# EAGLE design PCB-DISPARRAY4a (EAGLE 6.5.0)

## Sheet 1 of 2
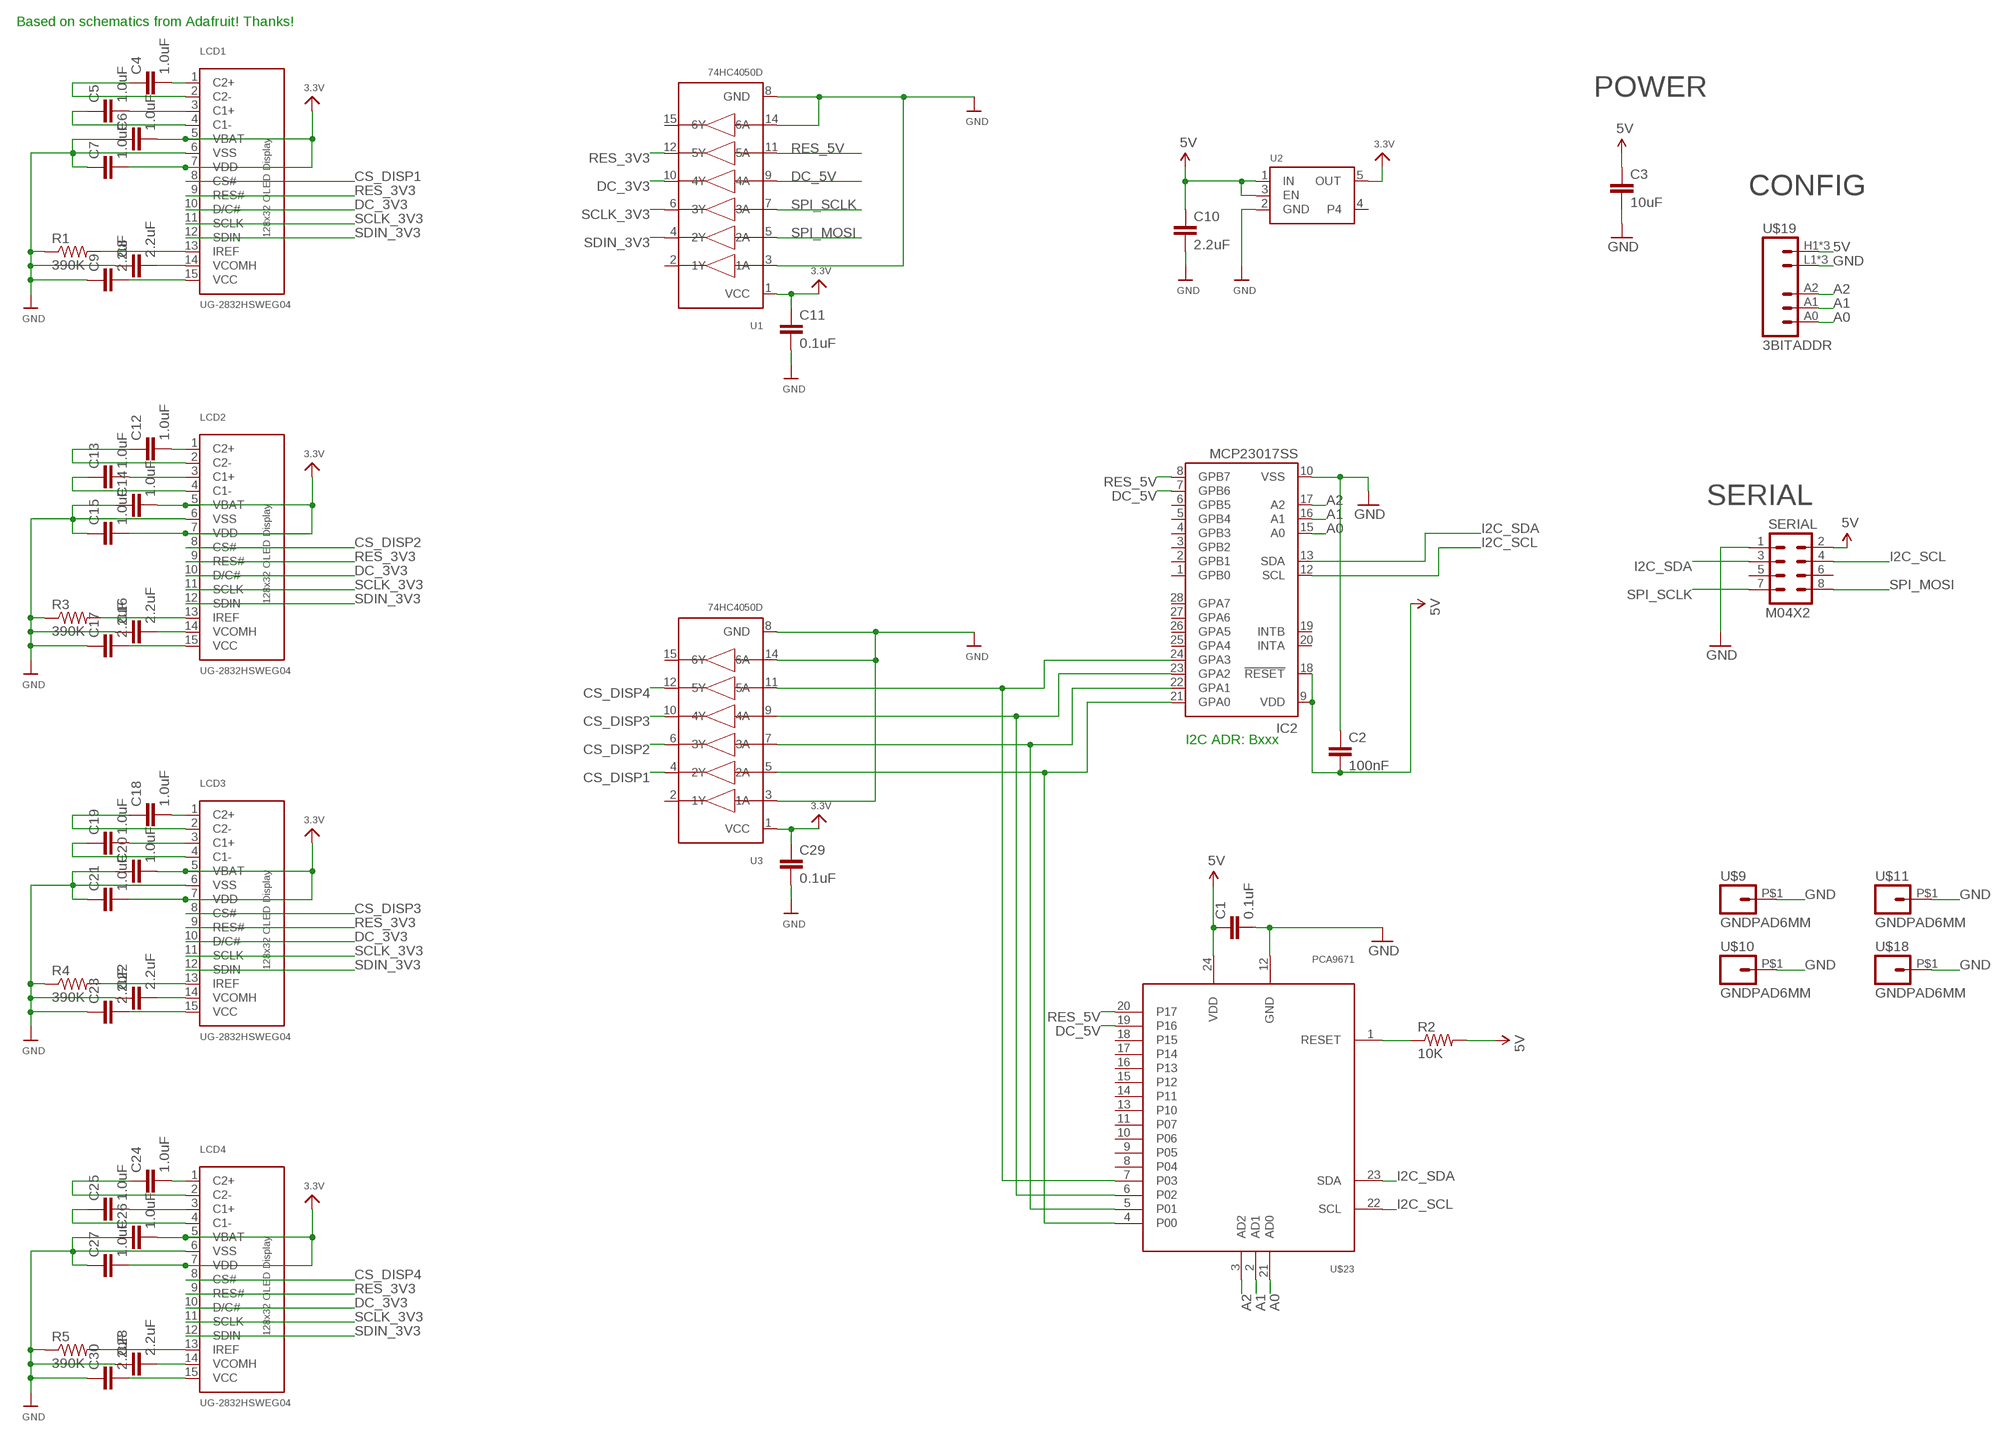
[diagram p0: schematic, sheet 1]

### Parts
C1  0.1uF  CAP0603-CAP  [0603-CAP]
C2  100nF  CAP0603-CAP  [0603-CAP]
C3  10uF  CAP0805  [0805]
C4  1.0uF  CAP0603-CAP  [0603-CAP]
C5  1.0uF  CAP0603-CAP  [0603-CAP]
C6  1.0uF  CAP0603-CAP  [0603-CAP]
C7  1.0uF  CAP0603-CAP  [0603-CAP]
C8  2.2uF  CAP0603-CAP  [0603-CAP]
C9  2.2uF  CAP0603-CAP  [0603-CAP]
C10  2.2uF  CAP0603-CAP  [0603-CAP]
C11  0.1uF  CAP0603-CAP  [0603-CAP]
C12  1.0uF  CAP0603-CAP  [0603-CAP]
C13  1.0uF  CAP0603-CAP  [0603-CAP]
C14  1.0uF  CAP0603-CAP  [0603-CAP]
C15  1.0uF  CAP0603-CAP  [0603-CAP]
C16  2.2uF  CAP0603-CAP  [0603-CAP]
C17  2.2uF  CAP0603-CAP  [0603-CAP]
C18  1.0uF  CAP0603-CAP  [0603-CAP]
C19  1.0uF  CAP0603-CAP  [0603-CAP]
C20  1.0uF  CAP0603-CAP  [0603-CAP]
C21  1.0uF  CAP0603-CAP  [0603-CAP]
C22  2.2uF  CAP0603-CAP  [0603-CAP]
C23  2.2uF  CAP0603-CAP  [0603-CAP]
C24  1.0uF  CAP0603-CAP  [0603-CAP]
C25  1.0uF  CAP0603-CAP  [0603-CAP]
C26  1.0uF  CAP0603-CAP  [0603-CAP]
C27  1.0uF  CAP0603-CAP  [0603-CAP]
C28  2.2uF  CAP0603-CAP  [0603-CAP]
C29  0.1uF  CAP0603-CAP  [0603-CAP]
C30  2.2uF  CAP0603-CAP  [0603-CAP]
IC2  MCP23017SS  [SSOP28]
LCD1  UG-2832HSWEG04  OLED_UG-2832HSWEG04WRAPAROUND  [UG-2832HSWEG04_WRAPAROUND]
LCD2  UG-2832HSWEG04  OLED_UG-2832HSWEG04WRAPAROUND  [UG-2832HSWEG04_WRAPAROUND]
LCD3  UG-2832HSWEG04  OLED_UG-2832HSWEG04WRAPAROUND  [UG-2832HSWEG04_WRAPAROUND]
LCD4  UG-2832HSWEG04  OLED_UG-2832HSWEG04WRAPAROUND  [UG-2832HSWEG04_WRAPAROUND]
R1  390K  RESISTOR0603-RES  [0603-RES]
R2  10K  RESISTOR0603-RES  [0603-RES]
R3  390K  RESISTOR0603-RES  [0603-RES]
R4  390K  RESISTOR0603-RES  [0603-RES]
R5  390K  RESISTOR0603-RES  [0603-RES]
SERIAL  M04X2  [2X4]
U1  74HC4050D  [SOIC16]
U2  VREG_SOT23-5  [SOT23-5]
U3  74HC4050D  [SOIC16]
U$9  GNDPAD6MM  [3.2MMPAD6MM]
U$10  GNDPAD6MM  [3.2MMPAD6MM]
U$11  GNDPAD6MM  [3.2MMPAD6MM]
U$18  GNDPAD6MM  [3.2MMPAD6MM]
U$19  3BITADDR  [3BITADDR]
U$23  PCA9671  [TSSOP24]

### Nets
3.3V: C6.2 C7.2 C11.1 C14.2 C15.2 C20.2 C21.2 C26.2 C27.2 C29.1 LCD1.5(VBAT) LCD1.7(VDD) LCD2.5(VBAT) LCD2.7(VDD) LCD3.5(VBAT) LCD3.7(VDD) LCD4.5(VBAT) LCD4.7(VDD) U1.1(VCC) U2.5(OUT) U3.1(VCC)
5V [Power]: C1.1 C2.2 C3.1 C10.1 IC2.9(VDD) IC2.18(!RESET) R2.2 SERIAL.2 U2.1(IN) U2.3(EN) U$19.H1(VCC) U$19.H2(VCC) U$19.H3(VCC) U$23.24(VDD)
A0: IC2.15(A0) U$19.A0 U$23.21(AD0)
A1: IC2.16(A1) U$19.A1 U$23.2(AD1)
A2: IC2.17(A2) U$19.A2 U$23.3(AD2)
CS_DISP1: LCD1.8(CS#) U3.4(2Y)
CS_DISP2: LCD2.8(CS#) U3.6(3Y)
CS_DISP3: LCD3.8(CS#) U3.10(4Y)
CS_DISP4: LCD4.8(CS#) U3.12(5Y)
DC_3V3: LCD1.10(D/C#) LCD2.10(D/C#) LCD3.10(D/C#) LCD4.10(D/C#) U1.10(4Y)
DC_5V: IC2.7(GPB6) U1.9(4A) U$23.19(P16)
GND [Power]: C1.2 C2.1 C3.2 C6.1 C7.1 C8.1 C9.1 C10.2 C11.2 C14.1 C15.1 C16.1 C17.1 C20.1 C21.1 C22.1 C23.1 C26.1 C27.1 C28.1 C29.2 C30.1 IC2.10(VSS) LCD1.6(VSS) LCD2.6(VSS) LCD3.6(VSS) LCD4.6(VSS) R1.1 R3.1 R4.1 R5.1 SERIAL.1 U1.3(1A) U1.8(GND) U1.14(6A) U2.2(GND) U3.3(1A) U3.8(GND) U3.14(6A) U$9.P$1 U$10.P$1 U$11.P$1 U$18.P$1 U$19.L1(GND) U$19.L2(GND) U$19.L3(GND) U$23.12(GND)
I2C_SCL: IC2.12(SCL) SERIAL.4 U$23.22(SCL)
I2C_SDA: IC2.13(SDA) SERIAL.3 U$23.23(SDA)
N$1: R2.1 U$23.1(RESET)
N$2: C4.1 LCD1.2(C2-)
N$3: C4.2 LCD1.1(C2+)
N$4: C5.1 LCD1.4(C1-)
N$5: C12.1 LCD2.2(C2-)
N$6: C12.2 LCD2.1(C2+)
N$7: C5.2 LCD1.3(C1+)
N$8: LCD1.13(IREF) R1.2
N$9: C8.2 LCD1.14(VCOMH)
N$10: C13.1 LCD2.4(C1-)
N$11: C13.2 LCD2.3(C1+)
N$12: LCD2.13(IREF) R3.2
N$13: C16.2 LCD2.14(VCOMH)
N$14: C17.2 LCD2.15(VCC)
N$15: C18.1 LCD3.2(C2-)
N$16: C18.2 LCD3.1(C2+)
N$17: C19.1 LCD3.4(C1-)
N$18: C19.2 LCD3.3(C1+)
N$19: LCD3.13(IREF) R4.2
N$20: C22.2 LCD3.14(VCOMH)
N$21: C23.2 LCD3.15(VCC)
N$22: C24.1 LCD4.2(C2-)
N$23: C24.2 LCD4.1(C2+)
N$24: C25.1 LCD4.4(C1-)
N$25: C25.2 LCD4.3(C1+)
N$26: LCD4.13(IREF) R5.2
N$27: C28.2 LCD4.14(VCOMH)
N$28: C9.2 LCD1.15(VCC)
N$29: IC2.21(GPA0) U3.5(2A) U$23.4(P00)
N$30: IC2.22(GPA1) U3.7(3A) U$23.5(P01)
N$31: IC2.23(GPA2) U3.9(4A) U$23.6(P02)
N$32: IC2.24(GPA3) U3.11(5A) U$23.7(P03)
N$33: C30.2 LCD4.15(VCC)
RES_3V3: LCD1.9(RES#) LCD2.9(RES#) LCD3.9(RES#) LCD4.9(RES#) U1.12(5Y)
RES_5V: IC2.8(GPB7) U1.11(5A) U$23.20(P17)
SCLK_3V3: LCD1.11(SCLK) LCD2.11(SCLK) LCD3.11(SCLK) LCD4.11(SCLK) U1.6(3Y)
SDIN_3V3: LCD1.12(SDIN) LCD2.12(SDIN) LCD3.12(SDIN) LCD4.12(SDIN) U1.4(2Y)
SPI_MOSI: SERIAL.8 U1.5(2A)
SPI_SCLK: SERIAL.7 U1.7(3A)
Unconnected: IC2.1(GPB0) IC2.2(GPB1) IC2.3(GPB2) IC2.4(GPB3) IC2.5(GPB4) IC2.6(GPB5) IC2.19(INTB) IC2.20(INTA) IC2.25(GPA4) IC2.26(GPA5) IC2.27(GPA6) IC2.28(GPA7) SERIAL.5 SERIAL.6 U1.2(1Y) U1.15(6Y) U2.4 U3.2(1Y) U3.15(6Y) U$23.8(P04) U$23.9(P05) U$23.10(P06) U$23.11(P07) U$23.13(P10) U$23.14(P11) U$23.15(P12) U$23.16(P13) U$23.17(P14) U$23.18(P15)

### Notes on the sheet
- Based on schematics from Adafruit! Thanks!
- POWER
- CONFIG
- SERIAL
- I2C ADR: Bxxx

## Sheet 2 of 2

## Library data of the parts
C1-C30 = SparkFun:CAP: Capacitor
IC2 = microchip:MCP23017: http://ww1.microchip.com/downloads/en/DeviceDoc/21952a.pdf Source: http://ww1.microchip.com/downloads/en/DeviceDoc/21952a.pdf; MF: MICROCHIP; MPN: MCP23017-E/SS; OC_FARNELL: 1467674; OC_NEWARK: 31K2960
LCD1-LCD4 = microbuilder:OLED_UG-2832HSWEG04: 128x32 SPI 0.91" Monochrome OLED Display
R1-R5 = SparkFun:RESISTOR: Resistor
SERIAL = SparkFun:M04X2
U1 U3 = microbuilder:74HC4050D: 6-channel level shifter 74HC4050D - 2V-6V Supply Digikey: 74HC4050D,653-ND Mouser: 771-74HC4050D-T
U2 = microbuilder:VREG_SOT23-5: SOT23-5 Fixed Voltage Regulators To better organise some of the SOT23-5 fixed voltage regulators in this library, this new part was created. Part Current Out V Out V In V Dropout Digikey Part No. ADP121 150mA 3.3V 3.4-5.5V 0.09V @ 150mA ADP121-AUJZ33R7CT-ND ADP121 150mA 3.0V 3.1-5.5V 0.09V @ 150mA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
U$9-U$11 U$18 = SKAARHOJ:GNDPAD
U$19 = SKAARHOJ:3BITADDR
U$23 = SKAARHOJ:PCA9671

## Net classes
0 default: width 0.203 mm, drill 0.406 mm, clearance 0.203 mm
1 Power: width 0.406 mm, drill 0.61 mm, clearance 0.203 mm
2 RELAY LINES: width 0.305 mm, drill 0.406 mm, clearance 0.254 mm
3 INput lines: width 0.203 mm, drill 0.406 mm, clearance 0.254 mm

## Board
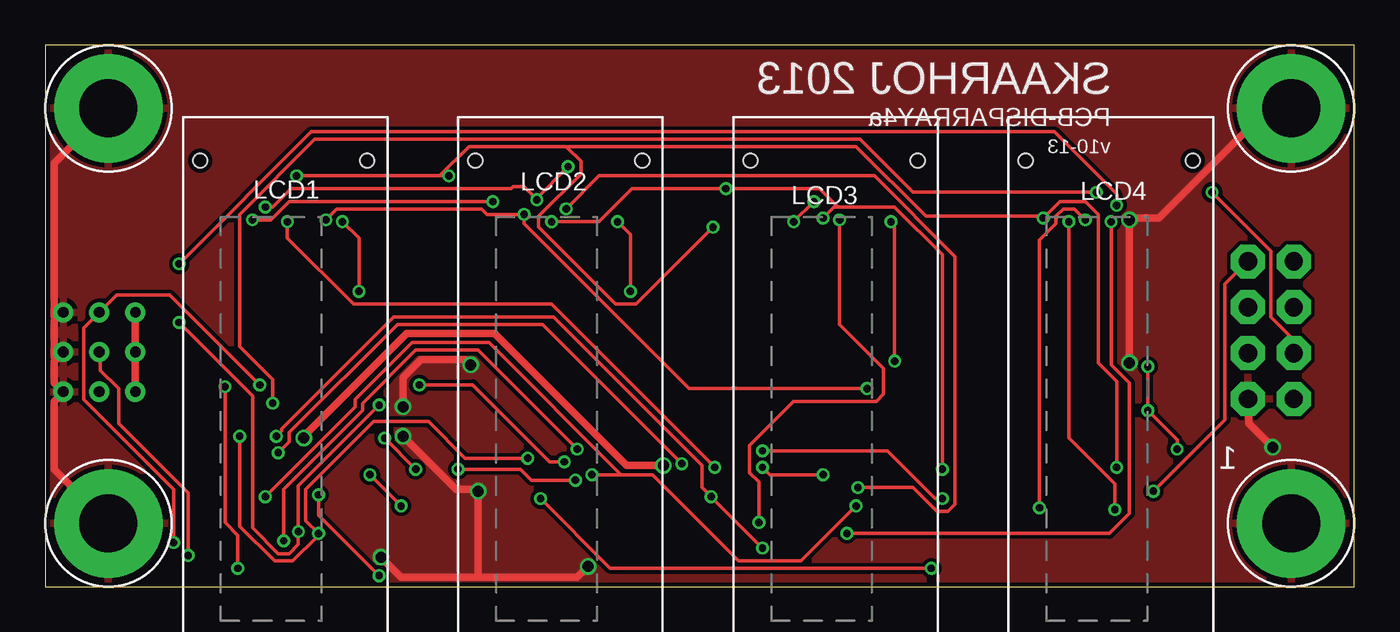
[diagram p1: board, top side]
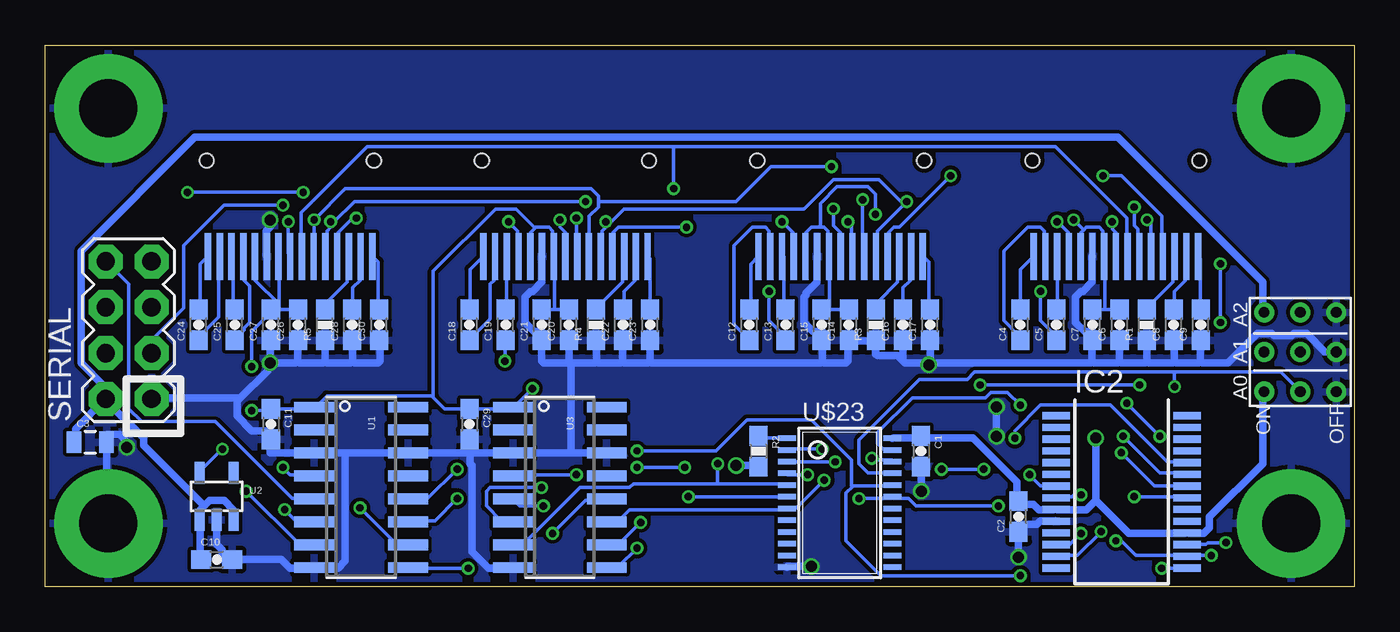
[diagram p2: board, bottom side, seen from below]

Size 72.5 x 30 mm. Coordinates in mm from the lower left corner, seen from the top.
Outline: 72.5,0 72.5,30 0,30 0,0 72.5,0
Copper layers (1*16): Top 0.035mm / dielectric 1.5mm / Bottom 0.035mm
Design rules "Fusion_eagle_rule_v1.1": minimum track width 6mil, minimum drill 12mil, track to track 6mil, track to pad 6mil, pad to pad 6mil, via to via 6mil, smd to smd 0mil, copper to edge 10mil, drill to drill 10mil, minimum pad ring 10mil, minimum via ring 6mil, stop-mask expansion 2mil, vias tented up to drill 100mil, thermal gap 10mil

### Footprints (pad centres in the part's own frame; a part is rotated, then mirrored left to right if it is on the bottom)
0603-CAP = smd 1.1 x 1: 1 -0.85,0; 2 0.85,0
0805 = smd 0.8 x 1.2: 1 -0.9,0; 2 0.9,0
SSOP28 = smd 0.4 x 1.5: 1 -4.225,-3.625; 2 -3.575,-3.625; 3 -2.925,-3.625; 4 -2.275,-3.625; 5 -1.625,-3.625; 6 -0.975,-3.625; 7 -0.325,-3.625; 8 0.325,-3.625; 9 0.975,-3.625; 10 1.625,-3.625; 11 2.275,-3.625; 12 2.925,-3.625; 13 3.575,-3.625; 14 4.225,-3.625; 15 4.225,3.625; 16 3.575,3.625; 17 2.925,3.625; 18 2.275,3.625; 19 1.625,3.625; 20 0.975,3.625; 21 0.325,3.625; 22 -0.325,3.625; 23 -0.975,3.625; 24 -1.625,3.625; 25 -2.275,3.625; 26 -2.925,3.625; 27 -3.575,3.625; 28 -4.225,3.625
UG-2832HSWEG04_WRAPAROUND = smd 2.6 x 0.35 bottom: 1 -7.7,-4.55; 2 -7.7,-3.9; 3 -7.7,-3.25; 4 -7.7,-2.6; 5 -7.7,-1.95; 6 -7.7,-1.3; 7 -7.7,-0.65; 8 -7.7,0; 9 -7.7,0.65; 10 -7.7,1.3; 11 -7.7,1.95; 12 -7.7,2.6; 13 -7.7,3.25; 14 -7.7,3.9; 15 -7.7,4.55 | hole 0.8: -2.4,4.625; -2.4,-4.625
0603-RES = smd 1.1 x 1: 1 -0.85,0; 2 0.85,0
2X4 = drill 1.016 pad 1.88 octagon: 1 -3.81,-1.27; 2 -3.81,1.27; 3 -1.27,-1.27; 4 -1.27,1.27; 5 1.27,-1.27; 6 1.27,1.27; 7 3.81,-1.27; 8 3.81,1.27
SOIC16 = smd 0.6 x 2.2: 1 -4.445,-2.6; 2 -3.175,-2.6; 3 -1.905,-2.6; 4 -0.635,-2.6; 5 0.635,-2.6; 6 1.905,-2.6; 7 3.175,-2.6; 8 4.445,-2.6; 9 4.445,2.6; 10 3.175,2.6; 11 1.905,2.6; 12 0.635,2.6; 13 -0.635,2.6; 14 -1.905,2.6; 15 -3.175,2.6; 16 -4.445,2.6
SOT23-5 = smd 0.55 x 1.2: 1 -0.95,-1.3; 2 0,-1.3; 3 0.95,-1.3; 4 0.95,1.3; 5 -0.95,1.3
3.2MMPAD6MM = drill 3.2 pad 6: P$1 0,0
3BITADDR = drill 0.6: A0 -2.2,0; A1 0,0; A2 2.2,0; H1 -2.2,2; H2 0,2; H3 2.2,2; L1 -2.2,-2; L2 0,-2; L3 2.2,-2
TSSOP24 = smd 0.305 x 0.991: 1 -4.225,-2.918; 2 -3.575,-2.918; 3 -2.925,-2.918; 4 -2.275,-2.918; 5 -1.625,-2.918; 6 -0.975,-2.918; 7 -0.325,-2.918; 8 0.325,-2.918; 9 0.975,-2.918; 10 1.625,-2.918; 11 2.275,-2.918; 12 2.925,-2.918; 13 2.925,2.918; 14 2.275,2.918; 15 1.625,2.918; 16 0.975,2.918; 17 0.325,2.918; 18 -0.325,2.918; 19 -0.975,2.918; 20 -1.625,2.918; 21 -2.275,2.918; 22 -2.925,2.918; 23 -3.575,2.918; 24 -4.225,2.918

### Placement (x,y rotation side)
C1  24,7.5 270 bottom
C2  18.6,3.89 90 bottom
C3  70,8 0 bottom
C4  18.5,14.5 90 bottom
C5  16.5,14.5 90 bottom
C6  13,14.5 90 bottom
C7  14.5,14.5 90 bottom
C8  10,14.5 90 bottom
C9  8.5,14.5 90 bottom
C10  63,1.5 0 bottom
C11  60,9 270 bottom
C12  33.5,14.5 90 bottom
C13  31.5,14.5 90 bottom
C14  28,14.5 90 bottom
C15  29.5,14.5 90 bottom
C16  25,14.5 90 bottom
C17  23.5,14.5 90 bottom
C18  49,14.5 90 bottom
C19  47,14.5 90 bottom
C20  43.5,14.5 90 bottom
C21  45,14.5 90 bottom
C22  40.5,14.5 90 bottom
C23  39,14.5 90 bottom
C24  64,14.5 90 bottom
C25  62,14.5 90 bottom
C26  58.5,14.5 90 bottom
C27  60,14.5 90 bottom
C28  55.5,14.5 90 bottom
C29  49,9 270 bottom
C30  54,14.5 90 bottom
IC2  12.89,5.25 270 bottom
LCD1  13.21,26 90 top
LCD2  28.45,26 90 top
LCD3  43.69,26 90 top
LCD4  58.93,26 90 top
R1  11.5,14.5 90 bottom
R2  33,7.5 270 bottom
R3  26.5,14.5 90 bottom
R4  42,14.5 90 bottom
R5  57,14.5 90 bottom
SERIAL  67.88,14.21 90 bottom
U1  55,5.5 270 bottom
U2  63,5 0 bottom
U3  44,5.5 270 bottom
U$9  69,3.5 0 top
U$10  3.5,3.5 0 top
U$11  69,26.5 0 top
U$18  3.5,26.5 0 top
U$19  3,13 90 bottom
U$23  28.5,4 270 bottom

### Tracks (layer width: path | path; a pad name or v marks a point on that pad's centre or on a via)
3.3V  (via drill 0.41)
  Top 0.203: v15.54,20.32 16.15,20.93 24.18,20.93 24.49,20.62 v26.52,20.62 26.52,20.12 35.66,10.97 v45.52,10.97 | v62.69,7.62 62.69,8.13 v61.06,9.75 v61.06,12.19
  Bottom 0.203: 13.82,15.34 14.43,15.34 C7.2 | 13.82,15.34 C6.2 | 13.82,15.34 13.82,18.29 LCD1.7 13.92,18.39 13.92,19.71 14.12,19.91 14.83,19.91 14.99,19.76 | 14.99,19.76 15.14,19.61 15.14,18.39 LCD1.5 | 29.06,15.34 29.46,15.34 C15.2 29.06,15.34 | 29.06,15.34 28.04,15.34 C14.2 | 29.06,15.34 29.06,18.29 LCD2.7 29.16,18.39 29.16,19.71 29.36,19.91 29.57,19.91 | 29.57,19.91 30.07,19.91 30.38,19.61 30.38,18.39 LCD2.5 | v15.54,20.32 14.99,19.76 | v26.52,20.62 26.52,21.74 26.92,22.15 28.65,22.15 29.57,21.23 29.57,19.91 | 59.54,15.34 59.94,15.34 C27.2 | 59.54,15.34 58.52,15.34 C26.2 | 59.54,15.65 59.54,18.29 LCD4.7 | 59.54,15.65 59.54,15.34 | 59.54,15.34 C27.2 | 59.54,15.65 60.86,16.97 60.86,18.29 LCD4.5 | 59.54,15.65 C27.2 | 44.3,15.34 44.91,15.34 C21.2 | 44.3,15.34 43.59,15.34 C20.2 | 44.3,15.34 44.3,18.29 LCD3.7 44.4,18.39 44.4,19.71 44.6,19.91 45.31,19.91 45.36,19.86 | 45.36,19.86 45.62,19.61 45.62,18.39 LCD3.5 | v62.69,7.62 63.91,6.4 U2.5 | v61.06,9.75 60.05,9.75 C11.1 59.94,9.86 57.61,9.86 U1.1 57.51,9.96 56.9,10.57 51.1,10.57 51.05,10.52 | 51.05,10.52 50.39,9.86 49.07,9.86 C29.1 48.97,9.86 46.63,9.86 U3.1 46.53,9.96 v45.52,10.97 | 45.36,19.86 46.43,20.93 47.55,20.93 51,17.48 51,10.57 51.05,10.52 | v61.06,12.19 61.06,14.12 59.94,15.24 C27.2
5V  (via drill 0.61)
  Top 0.406: U$19.H1 4.98,10.87 4.98,12.9 U$19.H2 4.98,13.21 4.98,15.14 U$19.H3 | v34.24,6.71 32.21,6.71 24.89,14.02 20.02,14.02 14.33,8.33 v14.33,8.23
  Bottom 0.406: C10.1 63.91,1.52 63.91,3.66 U2.1 63.91,3.86 63.91,4.27 63.7,4.47 | 63.7,4.47 63.4,4.78 62.59,4.78 62.08,4.27 62.08,3.76 U2.3 | C3.1 70.81,8.03 70.81,8.74 69.19,10.36 SERIAL.2 | 63.7,4.47 67.06,7.82 67.06,8.23 69.09,10.26 SERIAL.2 | U$23.24 25.5,8.23 24.18,8.23 24.08,8.33 C1.1 23.88,8.23 21.13,8.23 18.69,5.79 18.69,4.78 C2.2 18.49,4.57 17.78,4.57 17.48,4.27 16.66,4.27 IC2.9 16.46,4.27 14.83,4.27 14.33,4.78 | v34.24,6.71 33.02,6.71 R2.2 | 14.33,4.78 v14.33,8.23 | 14.33,4.78 12.5,2.95 9.35,2.95 IC2.18 9.14,2.95 8.33,2.95 8.03,3.25 8.03,3.86 5.08,6.81 5.08,10.77 U$19.H1 | SERIAL.2 69.19,10.57 69.19,11.07 70.51,12.39 70.51,18.59 64.21,24.89 13.11,24.89 5.08,16.87 5.08,15.24 U$19.H3
A0  (via drill 0.41)
  Top 0.203: v10.67,1.02 10.67,2.85 9.96,3.56 v9.96,11.07
  Bottom 0.203: 9.96,11.89 4.06,11.89 3.05,10.87 U$19.A0 | 9.96,11.89 21.03,11.89 21.44,11.48 24.08,11.48 27.43,8.13 27.43,6.81 26.92,6.3 25.6,6.3 U$23.21 | v10.67,1.02 9.35,1.02 IC2.15 | 9.96,11.89 v9.96,11.07
A1  (via drill 0.41)
  Top 0.203: v29.46,7.62 23.98,13.11 20.52,13.11 17.58,10.16 17.58,9.75 13.21,5.38 v13.21,2.54 | v7.92,1.73 7.92,5.18 4.06,9.04 4.06,10.97 3.05,11.99 3.05,12.9 U$19.A1
  Bottom 0.203: v29.46,7.62 31.39,7.62 U$23.2 | v13.21,2.54 12.9,2.54 12.09,1.73 9.35,1.73 IC2.16 9.25,1.73 v7.92,1.73
A2  (via drill 0.41)
  Top 0.203: v28.75,6.91 27.94,6.91 23.67,11.18 v20.73,11.18 | v11.89,11.18 6.91,16.15 3.96,16.15 3.05,15.24 U$19.A2 2.95,15.14 2.13,14.33 2.13,10.36 7.11,5.38 v7.11,2.44
  Bottom 0.203: v28.75,6.91 31.39,6.91 U$23.3 | v11.89,11.18 v20.73,11.18 | v7.11,2.44 8.13,2.44 8.23,2.34 9.25,2.34 IC2.17
CS_DISP1  (via drill 0.41)
  Top 0.203: v43.08,6.2 40.13,6.2 v39.73,6.6 | v37.08,6.6 28.04,15.65 17.07,15.65 13.41,19.3 v13.41,20.22
  Bottom 0.203: v43.08,6.2 46.53,6.2 U3.4 | v37.08,6.6 v39.73,6.6 | v13.41,20.22 13.41,19.81 13.21,19.61 LCD1.8
CS_DISP2  (via drill 0.41)
  Top 0.203: v45.01,5.49 48.06,5.49 49.38,4.17 49.99,4.17 50.39,4.57 50.39,18.29 45.92,22.76 30.68,22.76 v28.85,20.93
  Bottom 0.203: v45.01,5.49 47.85,5.49 48.06,5.28 48.06,4.47 47.24,3.66 46.63,3.66 U3.6 | v28.85,20.93 28.85,20.02 28.45,19.61 LCD2.8
CS_DISP3  (via drill 0.41)
  Top 0.203: v39.52,3.56 39.52,5.79 39.01,6.3 39.01,7.82 41.45,10.26 46.02,10.26 46.43,10.67 46.43,12.09 43.99,14.53 v43.99,20.32
  Bottom 0.203: v39.52,3.56 40.74,2.34 41.35,2.34 U3.10 | v43.99,20.32 43.99,19.91 43.69,19.61 LCD3.8
CS_DISP4  (via drill 0.41)
  Top 0.203: v44.4,2.95 58.93,2.95 60.05,4.06 60.05,11.28 59.03,12.29 v59.03,20.22
  Bottom 0.203: v44.4,2.95 42.57,4.78 41.45,4.78 U3.12 | v59.03,20.22 59.03,18.49 58.93,18.39 LCD4.8
DC_3V3  (via drill 0.41)
  Top 0.203: v12.19,21.03 12.6,21.03 13.61,22.05 25.81,22.05 25.91,22.15 26.52,22.15 v27.23,21.44 27.23,21.54 v28.96,23.27 | v55.07,4.37 55.07,19.2 55.98,20.12 55.98,20.52 56.39,20.93 57,20.93 v57.61,20.32
  Bottom 0.203: v12.19,21.03 12.19,20.02 11.99,19.81 11.99,18.39 LCD1.10 | v27.23,21.44 27.23,18.39 LCD2.10 | v55.07,4.37 53.03,2.34 52.43,2.34 U1.10 | LCD4.10 57.61,18.39 v57.61,20.32 55.88,22.05 42.27,22.05 41.86,21.64 41.86,21.34 | 41.86,21.34 41.86,21.03 42.37,20.52 42.37,18.39 LCD3.10 | v28.96,23.27 32.31,23.27 34.24,21.34 41.86,21.34
DC_5V  (via drill 0.41)
  Top 0.203: v17.98,6.2 v19.71,4.47 | v49.07,1.02 31.29,1.02 v27.43,4.88
  Bottom 0.203: v19.71,4.47 24.28,4.47 24.69,4.88 25.5,4.88 U$23.19 25.6,4.88 v27.43,4.88 | v17.98,6.2 17.37,5.59 16.56,5.59 IC2.7 | v49.07,1.02 52.32,1.02 U1.9
GND  (via drill 0.61)
  Top 0.406: 0.61,12.6 0.91,12.9 U$19.L2 | 0.61,12.6 0.51,12.5 0.51,11.28 0.91,10.87 U$19.L1 0.91,10.67 0.51,10.26 0.51,6.5 3.45,3.56 U$10.P$1 | 0.61,12.6 0.51,12.7 0.51,14.73 0.91,15.14 U$19.L3 0.51,14.94 0.51,23.47 3.45,26.42 U$18.P$1 | v30.07,1.12 29.46,0.51 23.98,0.51 | 23.98,0.51 19.71,0.51 v18.59,1.63 | 23.98,0.51 v23.98,5.28 23.88,5.38 22.76,5.38 v19.81,8.33 | v19.81,9.96 19.81,11.58 20.83,12.6 23.27,12.6 v23.57,12.29 | v67.97,7.72 66.65,9.04 66.65,10.36 SERIAL.1 | v60.05,12.39 v60.05,20.32 60.15,20.42 61.67,20.42 67.67,26.42 68.99,26.42 U$11.P$1
  Bottom 0.406: v30.07,1.12 31.39,1.12 U$23.12 | v18.59,1.63 18.59,2.95 C2.1 18.59,3.15 18.59,3.45 17.58,3.45 17.37,3.66 16.56,3.66 IC2.10 | v23.98,5.28 23.98,6.6 C1.2 | 8.53,12.5 8.53,13.61 C9.1 | 8.53,12.5 8.64,12.39 9.86,12.39 9.96,12.5 | 9.96,12.5 9.96,13.61 C8.1 | 11.48,12.5 11.48,13.61 R1.1 | 11.48,12.5 11.58,12.39 12.9,12.39 13.01,12.5 | 13.01,12.5 13.01,13.61 C6.1 | 14.53,12.5 14.53,13.61 C7.1 14.53,13.82 14.53,14.12 14.94,14.12 15.44,14.63 15.44,16.05 15.14,16.36 15.04,16.36 14.53,16.87 14.53,18.29 LCD1.6 | 14.53,12.5 14.43,12.39 13.11,12.39 13.01,12.5 | 9.96,12.5 10.06,12.39 11.38,12.39 11.48,12.5 | 29.46,12.5 29.36,12.39 28.14,12.39 28.04,12.5 28.04,13.61 C14.1 27.84,13.61 26.72,13.61 R3.1 26.52,13.61 26.52,12.9 26.42,12.8 25.3,12.8 24.99,12.5 | 29.46,12.5 29.46,13.61 C15.1 29.46,13.82 29.46,14.12 29.97,14.12 30.48,14.63 30.48,16.05 30.38,16.15 30.38,16.26 29.77,16.87 29.77,18.29 LCD2.6 | 23.47,12.5 23.47,13.61 C17.1 | 23.57,12.39 23.47,12.5 | 23.57,12.39 24.89,12.39 24.99,12.5 | 24.99,12.5 24.99,13.61 C16.1 | 14.53,12.5 14.63,12.39 23.37,12.39 23.47,12.5 | v19.81,9.96 v19.81,8.33 | v23.57,12.29 23.57,12.39 | v67.97,7.72 67.97,8.03 68.38,8.43 69.09,8.43 69.09,8.03 C3.2 69.09,7.82 69.09,3.56 U$9.P$1 | 55.47,12.5 55.37,12.39 54.05,12.39 53.95,12.5 53.95,13.61 C30.1 | 55.47,12.5 55.47,13.61 C28.1 | 57,12.5 57,13.61 R5.1 | 57,12.5 56.9,12.39 55.58,12.39 55.47,12.5 | 58.52,12.5 58.52,13.61 C26.1 | 58.52,12.5 58.42,12.39 57.1,12.39 57,12.5 | 60.05,12.5 60.05,13.61 C27.1 | 60.05,12.5 59.94,12.39 58.62,12.39 58.52,12.5 | v60.05,20.32 60.05,19.91 60.25,19.71 60.25,18.39 LCD4.6 | 60.05,12.5 v60.05,12.39 60.15,12.29 60.15,11.99 61.77,10.36
  Bottom 0.406: 39.01,12.5 39.01,13.61 C23.1 | 39.01,12.5 39.12,12.39 40.44,12.39 40.54,12.5 | 40.54,12.5 40.54,13.61 C22.1 | 41.96,12.5 41.96,13.61 R4.1 | 41.96,12.5 41.86,12.39 40.64,12.39 40.54,12.5 | 43.48,12.5 43.48,13.61 C20.1 | 43.38,12.39 43.48,12.5 | 43.38,12.39 42.06,12.39 41.96,12.5 | 43.48,12.5 43.59,12.39 44.91,12.39 45.01,12.5 45.01,13.61 C21.1 45.01,13.82 45.01,14.12 45.41,14.12 45.92,14.63 45.92,16.05 45.62,16.36 45.52,16.36 45.01,16.87 45.01,18.29 LCD3.6 | U2.2 62.99,3.66 62.99,2.34 62.69,2.03 62.69,1.52 62.18,1.52 C10.2 61.98,1.52 59.44,1.52 58.93,1.02 57.61,1.02 U1.8 57.4,1.02 56.29,1.02 55.88,1.42 55.88,7.42 | 48.97,7.42 48.97,8.13 C29.2 | 48.97,7.42 46.63,7.42 U3.3 46.43,7.42 43.38,7.42 | 43.38,7.42 41.45,7.42 U3.14 | 48.97,7.42 48.97,6.81 48.87,6.71 48.87,1.93 47.95,1.02 46.63,1.02 U3.8 | 48.97,7.42 52.32,7.42 U1.14 52.53,7.42 55.88,7.42 | 55.88,7.42 57.4,7.42 U1.3 60.05,7.42 60.05,8.13 C11.2 60.05,8.33 60.05,8.64 61.06,8.64 61.87,9.45 61.87,10.26 61.77,10.36 | 43.38,7.42 43.38,12.39 | SERIAL.1 66.55,10.46 61.87,10.46 61.77,10.36 | 29.46,12.5 29.57,12.39 38.91,12.39 39.01,12.5 | U$19.L2 1.02,13.01 1.63,13.01 2.64,14.02 3.35,14.02 3.45,13.92 4.47,13.92 4.57,14.02 5.38,14.02 7.01,12.39 8.43,12.39 8.53,12.5
  pour Top: 0,0 73,0 73,30 0,30
  pour Bottom: 0,0 73,0 73,30 0,30
I2C_SCL  (via drill 0.41)
  Top 0.203: v26.72,7.11 23.27,7.11 21.23,9.14 18.19,9.14 14.43,5.38 14.43,3.66 v15.14,2.95 15.04,2.95 15.04,2.74 13.72,1.42 12.7,1.42 10.77,3.35 v10.77,8.33 | v64.62,21.84 67.87,18.59 67.87,14.94 69.09,13.72 69.09,13.01 SERIAL.4 | v58.22,21.84 48.06,21.84 45.11,24.79 14.94,24.79 10.77,20.62 10.77,13.31 12.6,11.48 v12.6,10.16
  Bottom 0.203: v26.72,7.11 26.62,7.01 25.6,7.01 U$23.22 | v15.14,2.95 15.75,2.34 16.46,2.34 IC2.12 | v58.22,21.84 v64.62,21.84 | v10.77,8.33 v12.6,10.16
I2C_SDA  (via drill 0.41)
  Top 0.203: v18.49,10.06 14.02,5.59 v14.02,3.05 14.02,2.34 13.51,1.83 12.9,1.83 11.48,3.25 11.48,10.57 v7.42,14.63 | v59.33,21.13 59.33,21.74 55.88,25.2 14.73,25.2 v7.42,17.88
  Bottom 0.203: v18.49,10.06 19.2,10.77 20.12,10.77 20.42,10.46 24.49,10.46 26.42,8.53 26.42,7.92 26.11,7.62 25.6,7.62 U$23.23 | v14.02,3.05 15.34,1.73 16.46,1.73 IC2.13 | v59.33,21.13 62.59,21.13 64.82,18.9 64.82,15.44 66.55,13.72 66.55,13.01 SERIAL.3 | v7.42,14.63 v7.42,17.88
N$1
  Bottom 0.203: U$23.1 31.5,8.23 32.82,8.23 32.92,8.33 R2.1
N$2
  Bottom 0.203: C4.1 18.59,13.72 18.59,13.92 19.41,14.73 19.41,18.59 18.09,19.91 17.37,19.91 17.17,19.71 17.17,18.39 LCD1.2
N$3
  Bottom 0.203: C4.2 18.49,15.44 18.49,17.58 17.78,18.29 LCD1.1
N$4  (via drill 0.41)
  Top 0.203: v17.37,16.36 17.37,19.3 v16.46,20.22
  Bottom 0.203: v17.37,16.36 17.37,14.73 16.56,13.92 16.56,13.72 C5.1 | v16.46,20.22 15.85,19.61 15.85,18.39 LCD1.4
N$5
  Bottom 0.203: C12.1 33.53,13.72 34.34,14.53 34.34,18.9 33.33,19.91 32.61,19.91 32.41,19.71 32.41,18.39 LCD2.2
N$6
  Bottom 0.203: C12.2 33.43,15.44 33.43,17.88 33.02,18.29 LCD2.1
N$7
  Bottom 0.203: C5.2 16.46,15.44 16.46,18.29 LCD1.3
N$8
  Bottom 0.203: R1.2 11.48,15.44 10.06,16.87 10.06,18.29 LCD1.13
N$9
  Bottom 0.203: C8.2 9.96,15.44 9.96,16.36 9.35,16.97 9.35,18.29 LCD1.14
N$10  (via drill 0.41)
  Top 0.203: v32.41,16.36 32.41,19.51 v31.7,20.22
  Bottom 0.203: v32.41,16.36 32.41,14.73 31.6,13.92 31.6,13.72 C13.1 | v31.7,20.22 31.09,19.61 31.09,18.39 LCD2.4
N$11
  Bottom 0.203: C13.2 31.6,15.44 31.6,18.29 LCD2.3
N$12
  Bottom 0.203: R3.2 26.42,15.44 26.42,15.75 25.3,16.87 25.3,18.29 LCD2.13
N$13
  Bottom 0.203: C16.2 24.99,15.44 24.99,16.56 24.59,16.97 24.59,18.29 LCD2.14
N$14
  Bottom 0.203: C17.2 23.57,15.44 23.57,17.98 23.88,18.29 LCD2.15
N$15
  Bottom 0.203: C18.1 48.97,13.72 47.85,14.83 47.85,16.76 47.65,16.97 47.65,18.29 LCD3.2
N$16
  Bottom 0.203: C18.2 48.97,15.44 48.97,17.58 48.26,18.29 LCD3.1
N$17  (via drill 0.41)
  Top 0.203: v47.04,12.5 47.04,20.02 v46.84,20.22
  Bottom 0.203: v47.04,12.5 47.04,13.61 C19.1 | v46.84,20.22 46.33,19.71 46.33,18.39 LCD3.4
N$18
  Bottom 0.203: C19.2 46.94,15.44 46.94,18.29 LCD3.3
N$19
  Bottom 0.203: R4.2 41.96,15.44 40.54,16.87 40.54,18.29 LCD3.13
N$20
  Bottom 0.203: C22.2 40.44,15.44 40.44,16.36 39.83,16.97 39.83,18.29 LCD3.14
N$21
  Bottom 0.203: C23.2 39.01,15.44 39.01,18.19 39.12,18.29 LCD3.15
N$22
  Bottom 0.203: C24.1 63.91,13.72 63.91,13.92 62.89,14.94 62.89,18.29 LCD4.2
N$23
  Bottom 0.203: C24.2 63.91,15.44 63.91,17.88 63.5,18.29 LCD4.1
N$24
  Bottom 0.203: C25.1 61.98,13.72 61.47,14.22 61.47,14.33 61.16,14.63 61.16,16.66 61.47,16.97 61.47,18.29 LCD4.4
N$25
  Bottom 0.203: C25.2 62.08,15.44 62.08,18.29 LCD4.3
N$26
  Bottom 0.203: R5.2 57,15.44 57,15.65 55.78,16.87 55.78,18.29 LCD4.13
N$27
  Bottom 0.203: C28.2 55.47,15.44 55.47,16.56 55.07,16.97 55.07,18.29 LCD4.14
N$28
  Bottom 0.203: C9.2 8.53,15.44 8.53,18.19 8.64,18.29 LCD1.15
N$29  (via drill 0.41)
  Top 0.203: 31.9,6.2 33.63,6.2 38.41,1.42 41.86,1.42 v44.91,4.47 | 31.9,6.2 v30.28,6.2 | v12.19,4.98 17.17,9.96 17.17,10.36 20.32,13.51 24.59,13.51 31.9,6.2
  Bottom 0.203: v30.28,6.2 31.39,6.2 U$23.4 | v44.91,4.47 46.23,4.47 46.53,4.78 U3.5 | v12.19,4.98 9.35,4.98 IC2.21
N$30  (via drill 0.41)
  Top 0.203: v12.9,7.42 13.51,8.03 13.51,8.53 19.51,14.53 27.53,14.53 v35.26,6.81
  Bottom 0.203: 35.26,5.69 39.93,5.69 40.13,5.49 42.88,5.49 46.02,2.34 46.53,2.34 U3.7 | 35.26,5.69 31.5,5.69 U$23.5 | v12.9,7.42 11.07,5.59 9.35,5.59 IC2.22 | 35.26,5.69 v35.26,6.81
N$31  (via drill 0.41)
  Top 0.203: v39.73,2.13 v36.88,4.98 36.37,5.49 36.37,6.71 28.14,14.94 19.3,14.94 13.11,8.74 13.11,8.64 v12.8,8.33
  Bottom 0.203: v36.88,4.98 31.5,4.98 U$23.6 | v39.73,2.13 40.74,1.12 41.35,1.12 U3.9 | v12.8,8.33 10.77,6.3 9.35,6.3 IC2.23
N$32  (via drill 0.41)
  Top 0.203: v20.52,6.5 v18.8,8.23 | v22.86,6.5 26.31,6.5 26.92,5.89 v29.36,5.89
  Bottom 0.203: U3.11 41.35,3.66 40.74,3.66 40.13,4.27 31.5,4.27 U$23.7 31.39,4.37 30.89,4.37 v29.36,5.89 | v18.8,8.23 18.8,8.64 17.37,10.06 13.51,10.06 10.36,6.91 9.35,6.91 IC2.24 | v22.86,6.5 v20.52,6.5
N$33
  Bottom 0.203: C30.2 54.05,15.44 54.05,17.98 54.36,18.29 LCD4.15
RES_3V3  (via drill 0.41)
  Top 0.203: v49.68,6.5 49.68,18.39 47.04,21.03 43.89,21.03 | 43.89,21.03 43.69,21.03 v43.08,20.42 | v28.04,20.22 30.68,20.22 32.51,22.05 v37.69,22.05 42.88,22.05 43.89,21.03
  Bottom 0.203: v49.68,6.5 51.31,4.88 52.32,4.88 U1.12 | v43.08,20.42 43.08,18.39 LCD3.9 | v28.04,20.22 27.84,20.02 27.84,18.39 LCD2.9 | 37.69,24.38 54.66,24.38 58.32,20.73 58.32,18.39 LCD4.9 | 37.69,24.38 16.56,24.38 12.6,20.42 12.6,18.39 LCD1.9 | 37.69,24.38 v37.69,22.05
RES_5V  (via drill 0.41)
  Top 0.203: v18.49,0.61 15.14,3.96 v15.14,5.08 | v49.68,4.88 49.28,4.88 46.63,7.52 v39.73,7.52
  Bottom 0.203: 27.79,5.54 28.14,5.18 28.14,2.54 26.21,0.61 v18.49,0.61 | 27.79,5.54 27.74,5.59 25.6,5.59 U$23.20 | v15.14,5.08 15.54,5.08 15.65,4.98 16.46,4.98 IC2.8 | v49.68,4.88 50.9,3.66 52.32,3.66 U1.11 | v39.73,7.52 35.36,7.52 33.63,9.25 30.07,9.25 27.84,7.01 27.84,5.59 27.79,5.54
SCLK_3V3  (via drill 0.41)
  Top 0.203: v59.23,4.27 59.23,5.69 56.69,8.23 v56.69,20.22 | v11.48,20.32 12.5,20.32 13.51,21.34 v24.79,21.34 | v41.45,20.22 v42.57,21.34
  Bottom 0.203: v59.23,4.27 58.62,3.66 57.61,3.66 U1.6 | LCD4.11 56.9,18.39 56.9,19.71 56.69,19.91 v56.69,20.22 56.49,20.22 55.37,21.34 v42.57,21.34 | v11.48,20.32 11.28,20.12 11.28,18.39 LCD1.11 | LCD2.11 26.42,18.39 26.42,19.71 v24.79,21.34 24.99,21.23 26.31,22.55 28.85,22.55 30.48,20.93 40.44,20.93 41.3,20.07 | 41.3,20.07 41.66,19.71 41.66,18.39 LCD3.11 | 41.3,20.07 v41.45,20.22
SDIN_3V3  (via drill 0.41)
  Top 0.203: v59.33,6.6 59.33,11.38 58.32,12.39 58.32,20.62 57.61,21.34 56.19,21.34 v55.27,20.42 55.27,20.52 48.77,20.52 44.91,24.38 28.96,24.38 28.91,24.33 | v22.35,22.76 21.84,22.76 | 21.84,22.76 v13.92,22.76 | v36.98,19.91 32.72,15.65 31.6,15.65 27.33,19.91 27.33,20.52 29.67,22.86 29.67,23.57 28.91,24.33 | 28.91,24.33 28.85,24.38 23.47,24.38 21.84,22.76
  Bottom 0.203: v59.33,6.6 58.93,6.2 57.61,6.2 U1.4 | v55.27,20.42 55.47,20.42 56.29,19.61 56.29,18.39 LCD4.12 | v13.92,22.76 12.9,22.76 10.67,20.52 10.67,18.39 LCD1.12 | v22.35,22.76 25.2,19.91 25.5,19.91 25.81,19.61 25.81,18.39 LCD2.12 | v36.98,19.91 40.74,19.91 41.05,19.61 41.05,18.39 LCD3.12
SPI_MOSI
  Bottom 0.203: U1.5 58.83,4.88 63.09,9.14 67.16,9.14 67.87,9.86 67.87,16.76 69.09,17.98 SERIAL.8
SPI_SCLK  (via drill 0.41)
  Top 0.203: v61.37,5.28 65.33,9.25 65.33,16.76 66.55,17.98 SERIAL.7
  Bottom 0.203: v61.37,5.28 58.42,2.34 U1.7

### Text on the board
_tsilk: SKAARHOJ 2013 | PCB-DISPARRAY4a | v10-13 | 1

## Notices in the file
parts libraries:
SparkFun: Licensing: CC v3.0 Share-Alike You are welcome to use this library for commercial purposes.
